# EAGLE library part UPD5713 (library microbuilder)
UPD5713TK - Wide Band SPDT Switch (50MHz-2.5GHz) Digikey: UPD5713TK-E2-ACT-ND Mouser: 551-UPD5713TK-A
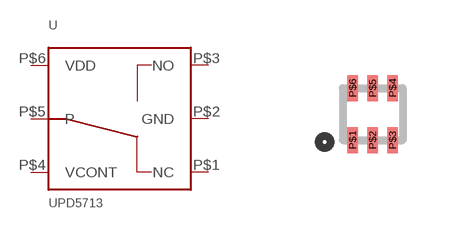
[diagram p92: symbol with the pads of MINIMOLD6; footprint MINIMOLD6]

Designator prefix U

## UPD5713  [MINIMOLD6]
P$1  NC
P$2  GND
P$3  NO
P$4  VCONT
P$5  P
P$6  VDD

## Footprint MINIMOLD6 (pad centres in mm)
6-Pin MINIMOLD Leadless Part Reference: http://www.cel.com/pdf/datasheets/upd5713tk.pdf
smd 0.26 x 0.65: P$1 -0.5,-0.65; P$2 0,-0.65; P$3 0.5,-0.65; P$4 0.5,0.65; P$5 0,0.65; P$6 -0.5,0.65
